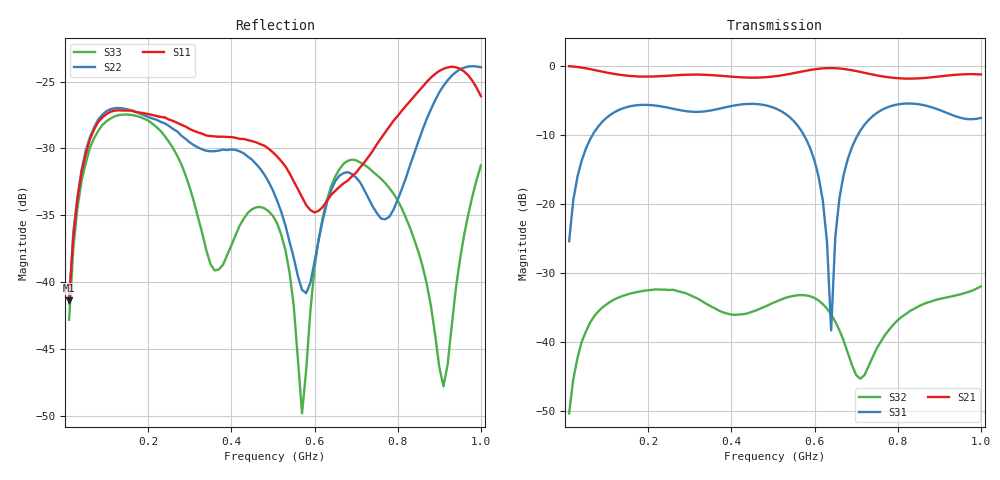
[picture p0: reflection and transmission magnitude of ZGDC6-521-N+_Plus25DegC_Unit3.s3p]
!Created: 04-01-2020 at 16:34:53
!Mini-Circuits
!S3P DATA File Format
!Type: Directional Coupler
!Port 1: (Input); Port 2: (Output); Port 3: (Couple)
!TEST CONDITIONS: Z:50 OHM SYSTEM, INPUT POWER = -10dBm, TEMP:25°C
!REMARK: Thru-Line loss normalized
!MODEL: ZGDC6-521-N+
!S/N: U3_25C
# MHZ S DB R 50
!Frequency
!  S11 dB  S11 DEG  S12 dB  S12 DEG  S13 dB  S13 DEG
!  S21 dB  S21 DEG  S22 dB  S22 DEG  S23 dB  S23 DEG
!  S31 dB  S31 DEG  S32 dB  S32 DEG  S33 dB  S33 DEG
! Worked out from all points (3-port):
!   100 points, 10 MHz to 1 GHz, reference 50 ohm
!   strongest paths, dB at 10 MHz, 260 MHz, 510 MHz, 760 MHz, 1 GHz:
!     S21: 0.0, -1.4, -1.5, -1.5, -1.2
!     S31: -25.4, -6.2, -6.2, -6.4, -7.5
!     S32: -50.3, -32.4, -34.1, -39.9, -31.9
!   lowest |S11| = -41.3 dB at 10 MHz (marker M1), VSWR 1.02, Z = 50.4 + j0.774 ohm
!   |S11| at or under -10 dB: start of sweep to end of sweep
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10  -41.35 63.8  -0.04 -7.5  -25.37 83.2
    -0.04 -7.5  -41.59 56.1  -51.81 -101.3
    -25.39 82.8  -50.32 -112.2  -42.80 68.4
130  -27.14 7.8  -1.27 -88.1  -6.37 15.1
     -1.27 -88.1  -26.97 -21.0  -33.52 94.5
     -6.37 15.1  -33.52 94.7  -27.50 2.8
280  -28.23 -17.2  -1.31 -179.0  -6.44 -34.7
     -1.31 -179.0  -29.04 -132.9  -32.77 -68.1
     -6.44 -34.7  -32.76 -67.9  -31.19 -47.5
510  -30.59 -36.1  -1.46 38.4  -6.25 -98.0
     -1.46 38.4  -33.89 -28.9  -34.06 111.4
     -6.25 -98.0  -34.09 111.2  -35.59 -45.3
570  -33.64 -33.3  -0.81 0.6  -9.55 -130.1
     -0.81 0.6  -40.58 -123.9  -33.18 50.8
     -9.55 -130.0  -33.19 50.9  -49.80 -149.8
640  -33.47 -4.4  -0.31 -49.0  -38.31 86.2
     -0.31 -49.0  -33.12 87.7  -36.00 -28.4
     -38.30 86.4  -35.98 -28.6  -32.82 65.4
680  -32.41 1.6  -0.52 -78.0  -13.50 -15.0
     -0.52 -78.0  -31.77 37.8  -41.56 -59.5
     -13.50 -15.0  -41.56 -59.6  -30.92 34.4
830  -26.45 -0.4  -1.84 -170.9  -5.44 -93.7
     -1.84 -170.9  -31.22 -168.0  -35.45 -99.4
     -5.45 -93.7  -35.49 -99.4  -35.96 -26.1
910  -24.04 -26.9  -1.46 140.9  -6.60 -119.4
     -1.46 140.9  -25.32 132.4  -33.61 -166.3
     -6.60 -119.4  -33.63 -166.3  -47.79 -132.2
1000  -26.08 -86.2  -1.24 81.0  -7.53 -126.8
      -1.24 81.0  -23.92 85.5  -31.95 126.4
      -7.53 -126.8  -31.94 126.4  -31.27 116.9
